TYPE "ST_CyclicRequest"
VERSION : 0.1


  STRUCT
   byServiceID : BYTE ;	//Service ID | 0x12 = Write/Read objects cyclic
   wDataLength : WORD ;	//Data length | Must be 0x15 in this request (Service ID, Data length, Acknowledg
   byAcknowledge : BYTE ;	//Acknowledge | Can be set to 0x00 in this request
   byMessageID : BYTE ;	//Message ID | Free usable message ID of the application | Can be set from the cl
   dwControlWord : DWORD ;	//Control word | Bit 0 = Manual mode | Bit 1 = Automatic mode | Bit 2 = Start hom
   byComMode : BYTE ;	//Communication mode | 0x00 = Acyclic communication mode | 0x01 = Cyclic communic
   diOffsetForceSensor : DINT ;	//Offset of the force sensor | Unit [N] 1 * 10^-2 (2 decimal places, e.g. 1 = 0,0
   byMotionMode : BYTE ;	//Motion mode (Jog, Move absolute/relative) | 0x00 = Jog | 0x01 = Move absolute |
   diMotionVelocity : DINT ;	//Motion velocity (Jog, Move absolute/relative) | Unit [mm/s] 1 * 10^-2 (2 decima
   diMotionPositionDistance : DINT ;	//Motion position/distance (Move absolute/relative) | Unit [mm] 1 * 10^-2 (2 deci
   wSelectedProgramNumber : WORD ;	//Selected program number
   byDigitalInputs : BYTE ;	//Digital inputs (Step enabling conditions in the sequencer of the press process)
  END_STRUCT ;
END_TYPE

